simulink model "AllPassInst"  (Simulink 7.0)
settings: Solver=ode45  StartTime=0.0  StopTime=10.0  RelTol=1e-6

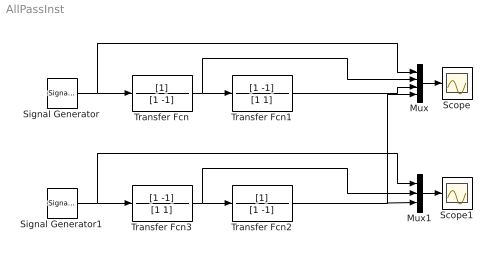
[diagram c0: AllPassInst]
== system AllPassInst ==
  Mux : Mux
  Mux1 : Mux  Inputs=3
  Scope : Scope
  Scope1 : Scope
  Signal Generator : SignalGenerator  WaveForm=square
  Signal Generator1 : SignalGenerator  WaveForm=square
  Transfer Fcn : TransferFcn  Denominator=[1 -1]
  Transfer Fcn1 : TransferFcn  Numerator=[1 -1]  Denominator=[1 1]
  Transfer Fcn2 : TransferFcn  Denominator=[1 -1]
  Transfer Fcn3 : TransferFcn  Numerator=[1 -1]  Denominator=[1 1]
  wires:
  Signal Generator/1 -> Transfer Fcn/1, Mux/1
  Transfer Fcn/1 -> Transfer Fcn1/1, Mux/2
  Mux/1 -> Scope/1
  Transfer Fcn1/1 -> Mux/3
  Signal Generator1/1 -> Mux1/1, Transfer Fcn3/1
  Transfer Fcn3/1 -> Mux1/2, Transfer Fcn2/1
  Mux1/1 -> Scope1/1
  Transfer Fcn2/1 -> Mux1/3, Mux/4
